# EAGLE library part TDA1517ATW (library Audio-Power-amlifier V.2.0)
8 W BTL or 2 ´ 4 W SE power amplifier
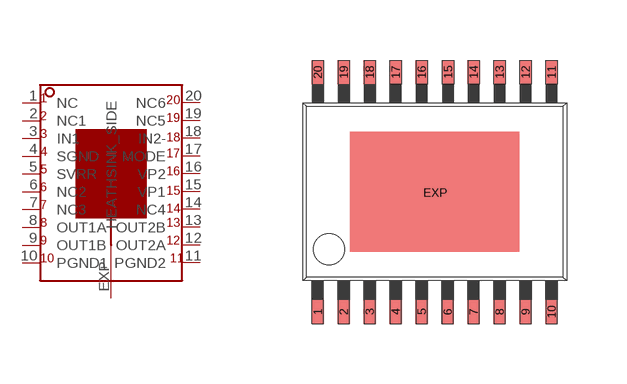
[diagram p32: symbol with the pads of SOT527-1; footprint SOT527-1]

Designator prefix IC

## TDA1517ATW  [SOT527-1]
1  NC  nc
2  NC1  nc
3  IN1  in
4  SGND  pwr
5  SVRR
6  NC2  nc
7  NC3  nc
8  OUT1A  out
9  OUT1B  out
10  PGND1  pwr
11  PGND2  pwr
12  OUT2A  out
13  OUT2B  out
14  NC4  nc
15  VP1  pwr
16  VP2  pwr
17  MODE
18  IN2-  in
19  NC5  nc
20  NC6  nc
EXP  HEATHSINK_SIDE  pwr

## Footprint SOT527-1 (pad centres in mm)
smd 0.305 x 0.61: 1 -2.925,-2.995; 2 -2.275,-2.995; 3 -1.625,-2.995; 4 -0.975,-2.995; 5 -0.325,-2.995; 6 0.325,-2.995; 7 0.975,-2.995; 8 1.625,-2.995; 9 2.275,-2.995; 10 2.925,-2.995; 11 2.925,2.995; 12 2.275,2.995; 13 1.625,2.995; 14 0.975,2.995; 15 0.335,2.995; 16 -0.325,2.995; 17 -0.975,2.995; 18 -1.625,2.995; 19 -2.275,2.995; 20 -2.925,2.995
smd 0.61 x 0.305: EXP 0.015,-0.015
